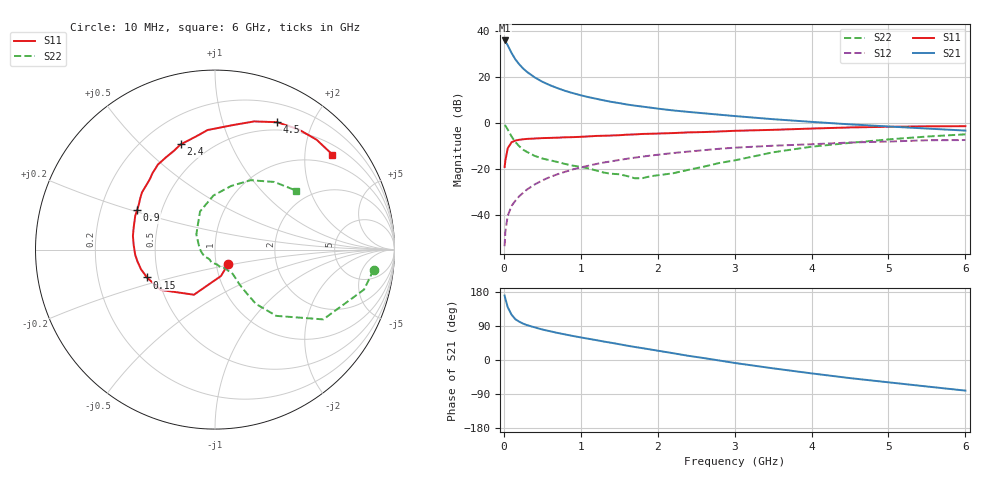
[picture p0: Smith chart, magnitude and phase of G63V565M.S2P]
! SIEMENS Small Signal Semiconductors
! BFG193
! Si NPN RF Bipolar Junction Transistor in SOT223
! VCE = 3.5 V  IC = 65 mA
! Common Emitter S-Parameters:  August  1996
# GHz  S  MA  R  50
!  f  S11  S21  S12  S22
! GHz  MAG  ANG  MAG  ANG  MAG  ANG  MAG  ANG
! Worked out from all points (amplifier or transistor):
!   36 points, 10 MHz to 6 GHz, reference 50 ohm
!   highest |S21| = 35.7 dB at 10 MHz (marker M1)
!   |S21| within 3 dB of that: start of sweep to 63.68 MHz
!   unconditionally stable (mu >= 1): 351.5 MHz to 2.363 GHz
!   at 250 MHz: K = 0.96, MSG = 27.0 dB, |S12| = -30.4 dB
!   at 1.4 GHz: K = 1.05, MAG = 11.5 dB, |S12| = -16.7 dB
!   at 6 GHz: K = 0.90, MSG = 2.1 dB, |S12| = -7.5 dB
!   S11 on the Smith chart (normalised r, x): 10 MHz: 1.14, -0.19; 150 MHz: 0.43, -0.16; 900 MHz: 0.36, +0.21; 2.4 GHz: 0.35, +0.66; 4.5 GHz: 0.40, +1.52; 6 GHz: 0.73, +2.65
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0.01  0.1095 -49.1  60.82 170.1  0.0021 83.8  0.8908 -7.3
0.02  0.1508 -77.2  58.05 161.7  0.0044 81.1  0.8599 -15.0
0.05  0.2774 -115.0  47.79 139.6  0.0095 72.4  0.7177 -32.8
0.1  0.377 -143.4  32.64 119.6  0.0157 69.0  0.5034 -47.2
0.15  0.4096 -157.7  23.64 107.6  0.0203 67.6  0.3791 -53.0
0.2  0.4268 -165.2  18.5 101.1  0.0254 69.8  0.3101 -53.9
0.25  0.4371 -171.4  15.03 96.0  0.0301 70.3  0.2602 -54.6
0.3  0.4453 -176.1  12.69 92.1  0.0355 71.1  0.2328 -54.8
0.4  0.454 176.7  9.643 86.2  0.0457 70.7  0.1911 -54.2
0.5  0.4635 170.6  7.746 80.5  0.0561 70.0  0.1674 -53.9
0.6  0.4683 165.8  6.501 75.9  0.0665 68.4  0.1532 -55.1
0.7  0.474 161.5  5.598 71.4  0.0765 67.2  0.1403 -57.7
0.9  0.4865 153.0  4.368 63.3  0.0974 63.1  0.1171 -61.7
1.1  0.5045 145.8  3.587 56.0  0.1168 59.7  0.1022 -72.7
1.3  0.5211 138.9  3.051 48.7  0.137 55.6  0.0828 -82.9
1.6  0.5502 129.3  2.485 37.9  0.1653 48.6  0.0699 -109.4
2.2  0.5959 112.6  1.847 17.9  0.22 34.8  0.08 -174.9
2.4  0.6167 108.1  1.715 11.0  0.2367 30.6  0.0951 163.0
3.5  0.7006 81.9  1.192 -22.0  0.3171 3.2  0.2283 111.4
4.5  0.7897 64.0  0.921 -47.8  0.3717 -16.9  0.3656 75.8
5.5  0.8338 47.2  0.747 -69.9  0.4163 -40.4  0.501 48.8
6  0.8414 39.0  0.675 -80.8  0.4209 -53.9  0.5597 35.9
